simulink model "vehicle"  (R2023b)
settings: Solver=ode3  StartTime=0.0  StopTime=t_end  FixedStep=dt8dof  RelTol=1e-3
PreLoadFcn:
  | define_swarm_buses(3, 1000);
model workspace (MAT data in the model file):
  Af = 1.8
  Cp_tyre = 500
  Cx = 0.28
  G = 15000
  Ha = 0.4
  Hg = 0.4
  Hroll = 0.304
  Hroll_f = 0.08
  Hroll_r = 0.12
  Ir = 0.8
  Ix = 450
  Jz = 1800
  K = 130000
  K_psi = 0.48
  K_y = 0.06
  Karb_F = 26000
  Karb_R = 26000
  KdF = 0
  KdR = 0
  Kd_h = 0
  Kd_v = 0
  Kd_y = 0
  Ki_h = 0
  Ki_v = 0.1
  Ki_y = 0
  Kp_h = 1.5
  Kp_v = 1.5
  Kp_y = 0.1
  Ks_f = 39000
  Ks_r = 39000
  Kv = 290000
  L = 1.5
  Lril_L = 0.055
  Lril_T = 0.5
  MAX_PATH_LEN = 1000
  Pacn = [3000 1 1 1 1 1 1 1 1 0 0 0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]
  R0 = 0.2
  Rfront = 0.2
  Rr_sterzo = 0
  Rrear = 0.2
  Rs = 13
  Tf = 1.5
  Tr = 1.5
  a = 0.6
  a_brake = -3
  b = 0.9
  camb_0F = 0
  camb_0R = -0.00680678408278
  d_max = 0.558505360638
  dt8dof = 0.002
  dtastar = 0.1
  dtcontrol = 0.03
  f0 = 0.0041
  f2 = 2.051e-07
  g = 9.81
  m = 1300
  mot_T_table = [0 0 0 0 0 0 0 0 0 0 0 0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]
  mot_alpha_bp = [0 10 20 30 40 50 60 70 80 90 100]
  mot_n_bp = [0 29.9163426864 59.8326853729 89.7490280593 119.665370746 149.581713432 179.498056119 209.414398805 239.330741492 269.247084178 299.163426864 329.079769551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]
  mpc_speed : object (value not decoded)
  phi_road0 = 0
  psi0 = 0
  r_goal = 5
  r_slow = 30
  replan_steps = 20
  rho = 1.3
  slope_x_body0 = 0
  slope_y_body0 = 0
  t_end = 70
  terrain_truth_mu_table = [-1 -1 -1 -1 -1 -1 -1 -1 -1 -1 -1 -1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]
  terrain_truth_obstacle_table = [1 1 1 1 1 1 1 1 1 1 1 1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]
  terrain_truth_slope_deg_table = [2.67415653197 2.67413215857 2.67406695826 2.6739952249 2.6739164067 2.67382991742 2.67373513563 2.67363140411 2.67351802953 2.67339428225 2.67325939642 2.67311257041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]
  terrain_truth_slope_x_table = [-0.0458815772305 -0.0458808922252 -0.0458794511544 -0.0458778616187 -0.0458761104845 -0.0458741837099 -0.0458720663111 -0.0458697423295 -0.0458671948025 -0.0458644057365 -0.0458613560839 -0.045858025724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]
  terrain_truth_slope_y_table = [0.00874081815183 0.00874213563744 0.00874360556 0.00874524373283 0.00874706738108 0.00874909524079 0.00875134766185 0.00875384671474 0.00875661630067 0.00875968226488 0.00876307251276 0.0087668171283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]
  terrain_truth_traversable_table = [0 0 0 0 0 0 0 0 0 0 0 0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]
  terrain_truth_x_bp = [0 1 2 3 4 5 6 7 8 9 10 11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]
  terrain_truth_y_bp = [0 1 2 3 4 5 6 7 8 9 10 11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]
  teta0 = 0
  tetapunto0 = 0
  theta_road0 = 0
  toe_F = -0.00174532925199
  toe_R = 0.00174532925199
  velstart = 5
  wr0_FL = 3.15
  wr0_FR = 3.15
  wr0_RL = 3.15
  wr0_RR = 3.15
  x0 = 0
  y0 = 0
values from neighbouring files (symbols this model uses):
  gear_ratio = 10    [motor_map.m]
  v_ref_init = scenario.vehicle8.velstart    [make_vref_filter.m]
undefined symbols (not defined in the file or in its folder): A_f, B_f, C_f, D_f, psi0_1
libraries: simulink_extras x15, mpclib x1, slpidlib x1
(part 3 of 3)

== matlab function vehicle/PLANT/VEHICLE 8DOF/Interazione 
Pneumatici-Terreno/Pneumatico FR/Calcolo FORZA LATERALE & LONGITUDINALE
(Pneumatico - Terreno)/Pacejka 96 ==
function [F_pac,C_F] = fcn(Pac,gamma,slip,alfa,Fz,mu,Vcx,R0)
% function x il calcolo delle forze Fx, Fy e Mz

% Pac   -> struttura con coeff. Pacejka 96
% slip     -> scorrimento
% alfa  -> deriva [rad]
% gamma -> camber [rad]
% Vcx,y componenti della velocita' del centro di contatto C della ruota

% Ricostruzione struttura: coefficienti modello 
Pa_FZ0_ = Pac(1);
Pa_LFZ0 = Pac(2);
Pa_LmuV = Pac(3);
Pa_LKXK = Pac(4);
Pa_LKYA = Pac(5);
Pa_LCX_ = Pac(6);
Pa_LCY_ = Pac(7);
Pa_LEX_ = Pac(8);
Pa_LEY_ = Pac(9);
Pa_LHX_ = Pac(10);
Pa_LHY_ = Pac(11);
Pa_LVX_ = Pac(12);
Pa_LVY_ = Pac(13);
Pa_LKYG = Pac(14);
Pa_LKZG = Pac(15);
Pa_LT__ = Pac(16);
Pa_MR__ = Pac(17);
Pa_LXA_ = Pac(18);
Pa_LYK_ = Pac(19);
Pa_LVYK = Pac(20);
Pa_LS__ = Pac(21);
Pa_LCZ_ = Pac(22);
Pa_LMX_ = Pac(23);
Pa_LMY_ = Pac(24);
Pa_PCX1 = Pac(25);
Pa_PDX1 = Pac(26);
Pa_PDX2 = Pac(27);
Pa_PEX1 = Pac(28);
Pa_PEX2 = Pac(29);
Pa_PEX3 = Pac(30);
Pa_PEX4 = Pac(31);
Pa_PKX1 = Pac(32);
Pa_PKX2 = Pac(33);
Pa_PKX3 = Pac(34);
Pa_PHX1 = Pac(35);
Pa_PHX2 = Pac(36);
Pa_PVX1 = Pac(37);
Pa_PVX2 = Pac(38);
Pa_RBX1 = Pac(39);
Pa_RBX2 = Pac(40);
Pa_RCX1 = Pac(41);
Pa_RHX1 = Pac(42);
Pa_RTX1 = Pac(43);
Pa_RTX2 = Pac(44);
Pa_RTX3 = Pac(45);
Pa_QSX1 = Pac(46);
Pa_QSX2 = Pac(47);
Pa_QSX3 = Pac(48);
Pa_PCY1 = Pac(49);
Pa_PDY1 = Pac(50);
Pa_PDY2 = Pac(51);
Pa_PDY3 = Pac(52);
Pa_PEY1 = Pac(53);
Pa_PEY2 = Pac(54);
Pa_PEY3 = Pac(55);
Pa_PEY4 = Pac(56);
Pa_PKY1 = Pac(57);
Pa_PKY2 = Pac(58);
Pa_PKY3 = Pac(59);
Pa_PHY1 = Pac(60);
Pa_PHY2 = Pac(61);
Pa_PHY3 = Pac(62);
Pa_PVY1 = Pac(63);
Pa_PVY2 = Pac(64);
Pa_PVY3 = Pac(65);
Pa_PVY4 = Pac(66);
Pa_RBY1 = Pac(67);
Pa_RBY2 = Pac(68);
Pa_RBY3 = Pac(69);
Pa_RCY1 = Pac(70);
Pa_RHY1 = Pac(71);
Pa_RVY1 = Pac(72);
Pa_RVY2 = Pac(73);
Pa_RVY3 = Pac(74);
Pa_RVY4 = Pac(75);
Pa_RVY5 = Pac(76);
Pa_RVY6 = Pac(77);
Pa_PTY1 = Pac(78);
Pa_PTY2 = Pac(79);
Pa_QSY1 = Pac(80);
Pa_QSY2 = Pac(81);
Pa_QBZ1 = Pac(82);
Pa_QBZ2 = Pac(83);
Pa_QBZ3 = Pac(84);
Pa_QBZ4 = Pac(85);
Pa_QBZ5 = Pac(86);
Pa_QBZ6 = Pac(87);
Pa_QBZ9 = Pac(88);
Pa_QBZZ = Pac(89);
Pa_QCZ1 = Pac(90);
Pa_QDZ1 = Pac(91);
Pa_QDZ2 = Pac(92);
Pa_QDZ3 = Pac(93);
Pa_QDZ4 = Pac(94);
Pa_QDZ6 = Pac(95);
Pa_QDZ7 = Pac(96);
Pa_QDZ8 = Pac(97);
Pa_QDZ9 = Pac(98);
Pa_QEZ1 = Pac(99);
Pa_QEZ2 = Pac(100);
Pa_QEZ3 = Pac(101);
Pa_QEZ4 = Pac(102);
Pa_QEZ5 = Pac(103);
Pa_QHZ1 = Pac(104);
Pa_QHZ2 = Pac(105);
Pa_QHZ3 = Pac(106);
Pa_QHZ4 = Pac(107);
Pa_SSZ1 = Pac(108);
Pa_SSZ2 = Pac(109);
Pa_SSZ3 = Pac(110);
Pa_SSZ4 = Pac(111);
Pa_QTZ1 = Pac(112);

% Costanti
epsi = 0.01;
eps_V = 0.1;
csi_0=1;
csi_4=1;
Amu = 10;
Pa_LmuX = mu;
Pa_LmuY = mu;

%-------------------------------- Fx pure slip ---------------------------
Cx = Pa_PCX1*Pa_LCX_;
dfz = (Fz-Pa_LFZ0*Pa_FZ0_)/(Pa_LFZ0*Pa_FZ0_);
mux = Pa_LmuX * (Pa_PDX1 + Pa_PDX2 * dfz);
Dx = mux*Fz; %*csi_1, con csi_1=1
%Shx = (Pa_PHX1+Pa_PHX2*dfz)*Pa_LHX_;
Shx = 0;
Kx = slip + Shx;
Ex = (Pa_PEX1+Pa_PEX2*dfz+Pa_PEX3*dfz^2)*(1-Pa_PEX4*sign(Kx))*Pa_LEX_;
if Ex>1 Et=1; end
Kxk = Fz*(Pa_PKX1+Pa_PKX2*dfz)*exp(Pa_PKX3*dfz)*Pa_LKXK;
Bx = Kxk/(Cx*Dx+epsi);
lam_mux  = Pa_LmuX*Amu/(1+(Amu-1)*Pa_LmuX);
SVx = Fz*(Pa_PVX1+Pa_PVX2*dfz)*(abs(Vcx)/(abs(Vcx)+eps_V))*Pa_LVX_*lam_mux; %*csi_1, con csi_1=1

% logitudinal slip stiffness (pendenza curva Fx nell'origine)
C_Fk = Bx*Cx*Dx;

% Forza longitudinale
Fx0 = Dx*sin(Cx*atan(Bx*Kx-Ex*(Bx*Kx-atan(Bx*Kx)))) + SVx;

%---------------------------- Fy pure side slip --------------------------
seg=sign(Vcx);
if seg==0 seg=1; end
alfa_star = tan(alfa)*seg;
gam_star = sin(gamma);
Shy = (Pa_PHY1+Pa_PHY2*dfz)*Pa_LHY_+Pa_PHY3*gam_star*Pa_LKYG*csi_0+csi_4-1;
alfa_y = alfa_star + Shy;
Cy = Pa_PCY1*Pa_LCY_;
muy = Pa_LmuY*(Pa_PDY1+Pa_PDY2*dfz)*(1-Pa_PDY3*gam_star^2);
Dy = muy*Fz; %*csi_2, con csi_2=1
Ey = (Pa_PEY1+Pa_PEY2*dfz)*(1-(Pa_PEY3+Pa_PEY4*gam_star)*sign(alfa_y))*Pa_LEY_;
if Ey>1 Ey=1; end
Kya0 = Pa_PKY1*Pa_LFZ0*Pa_FZ0_*sin(2*atan(Fz/(Pa_PKY2*Pa_LFZ0*Pa_FZ0_)))*Pa_LKYA;
Kya = Kya0*(1-Pa_PKY3*gam_star^2); %*csi_3, con csi_3=1
By = Kya/(Cy*Dy+epsi);
lam_muy = Pa_LmuY*Amu/(1+(Amu-1)*Pa_LmuY);
SVy = Fz*((Pa_PVY1+Pa_PVY2*dfz)*Pa_LVY_+(Pa_PVY3+Pa_PVY4*dfz)*gam_star*Pa_LKYG )*lam_muy; %*csi_2, con csi_2=1
Kyg0 = (Pa_PHY3*Kya0+Fz*(Pa_PVY3+Pa_PVY4*dfz))*Pa_LKYG;

% cornering stiffness (pendenza curva Fy nell'origine)
C_Fa = By*Cy*Dy;

% Forza laterale
Fy0 = Dy*sin(Cy*atan(By*alfa_y-Ey*(By*alfa_y-atan(By*alfa_y)))) + SVy;

% --------------------- Fx combined slip ------------------------------
Shxa = Pa_RHX1;
%Exa = Pa_REX1+Pa_REX2*dfz; NON esiste Pa.REX1 ne' Pa.REX2
Exa = 0;
Cxa = Pa_RCX1;
Bxa = Pa_RBX1*cos(atan(Pa_RBX2*slip))*Pa_LXA_;
alfaS = alfa_star+Shxa;
Gxa0 = cos(Cxa*atan(Bxa*Shxa-Exa*(Bxa*Shxa-atan(Bxa*Shxa))));
Gxa = cos(Cxa*atan(Bxa*alfaS-Exa*(Bxa*alfaS-atan(Bxa*alfaS))))/Gxa0;
Fx = Fx0*Gxa;

% ---------------------- Fy combined slip ------------------------------
Dvyk = muy*Fz*(Pa_RVY1+Pa_RVY2*dfz+Pa_RVY3*gam_star)*cos(atan(Pa_RVY4*alfa_star));%*csi_2, con csi_2=1
Svyk = Dvyk*sin(Pa_RVY5*atan(Pa_RVY6*slip));
Shyk = Pa_RHY1; %+Pa.RHY2*dfz; NON esiste Pa.RHY2
Cyk = Pa_RCY1;
Byk = Pa_RBY1*cos(atan(Pa_RBY2*(alfa_star-Pa_RBY3)))*Pa_LYK_;
%Eyk = Pa_REY1+Pa_REY2*dfz; NON esiste Pa.REY1 ne' Pa.REY2
Eyk = 0;
ks = slip+Shyk;
Gyk0 = cos(Cyk*atan(Byk*Shyk-Eyk*(Byk*Shyk-atan(Byk*Shyk))));
Gyk = cos(Cyk*atan(Byk*ks-Eyk*(Byk*ks-atan(Byk*ks))))/Gyk0;
Fy = Fy0*Gyk+Svyk;

% --------------------- Mz pure side slip  ---------------------------
Shf = Shy+SVy/Kya;
alfa_r = alfa_star+Shf;
Br = (Pa_QBZ9/Pa_LmuY+Pa_QBZZ*By*Cy); %*csi_6, con csi_6=1
%%% Pa_QBZZ e' in realta' QBZ10 scritto cosi' x ragioni di spazio
Cr = 1; %*csi_7, con csi_7=1
Dr = Fz*R0*((Pa_QDZ6+Pa_QDZ7*dfz)+(Pa_QDZ8+Pa_QDZ9*dfz)*gam_star)*cos(alfa)*Pa_LmuY*seg; %+csi_8-1, con csi_8=1
Mzr0 = Dr*cos(Cr*atan(Br*alfa_r));
Sht = Pa_QHZ1+Pa_QHZ2*dfz+(Pa_QHZ3+Pa_QHZ4*dfz)*gam_star;
alfa_t = alfa_star+Sht;
Bt = (Pa_QBZ1+Pa_QBZ2*dfz+Pa_QBZ3*dfz^2)*(1+Pa_QBZ5*abs(gam_star)+Pa_QBZ6*gam_star^2)*Pa_LKYA/Pa_LmuY;
if Bt<0 Bt=0; end
Ct = Pa_QCZ1;
Dt0 = Fz*R0/(Pa_LFZ0*Pa_FZ0_)*(Pa_QDZ1+Pa_QDZ2*dfz)*seg;
Dt = Dt0*(1+Pa_QDZ3*abs(gam_star)+Pa_QDZ4*gam_star^2); %*csi_5, con csi_5=1
Et = (Pa_QEZ1+Pa_QEZ2*dfz+Pa_QEZ3*dfz^2)*(1+(Pa_QEZ4+Pa_QEZ5*gam_star)*2/pi*atan(Bt*Ct*alfa_t));
if Et>1 Et=1; end
t0 = Dt*cos(Ct*atan(Bt*alfa_t - Et*(Bt*alfa_t-atan(Bt*alfa_t))))*cos(alfa);
Mz0 = -t0*Fy;
Kza0 = Dt0*Kya0;
%Kzg0 = Fz*R0*(Pa_QDZ8+Pa_QDZ9*dfz)-Dt0*Kyg0;

% momento autoallineamento (aligning torque)
Mz = Mz0 + Mzr0;

% ------------------------ Mz Combined -----------------------------
eps_k = 0; % ???????
lambda_s = Pa_LS__ ;
Fz0p = Pa_LFZ0*Pa_FZ0_;
K_yap = Kya + eps_k;
alfa_req = sqrt(alfa_r^2+(Kxk/K_yap)^2*slip^2)*sign(alfa_r);
alfa_teq = sqrt(alfa_t^2+(Kxk/K_yap)^2*slip^2)*sign(alfa_t);
s = R0*(Pa_SSZ1 + Pa_SSZ2*(Fy/Fz0p) + (Pa_SSZ3+Pa_SSZ4*dfz)*gam_star)*lambda_s;
Mzr = Dr*cos(Cr*atan(Br*alfa_req));
Fyp = Fy-Svyk; 
t = Dt*cos(Ct*atan(Bt*alfa_teq - Et*(Bt*alfa_teq-atan(Bt*alfa_teq))))*cos(alfa);
Mzp = -t*Fyp;
% momento autoallineamento (aligning torque)
Mz = Mzp + Mzr + s*Fx;
%%%%%%%%%%%%%%%%%%%%%%%

% Controllo che forza verticale Fz sia positiva
if Fz <= 0
    Fx = 0;
    Fy = 0;
    Mz = 0;
end

% Output
F_pac = [Fx; Fy; Mz];
C_F = [C_Fk; C_Fa];

== matlab function vehicle/PLANT/VEHICLE 8DOF/Interazione 
Pneumatici-Terreno/Pneumatico RL/Calcolo FORZA LATERALE & LONGITUDINALE
(Pneumatico - Terreno)/Pacejka 96 ==
function [F_pac,C_F] = fcn(Pac,gamma,slip,alfa,Fz,mu,Vcx,R0)
% function x il calcolo delle forze Fx, Fy e Mz

% Pac   -> struttura con coeff. Pacejka 96
% slip     -> scorrimento
% alfa  -> deriva [rad]
% gamma -> camber [rad]
% Vcx,y componenti della velocita' del centro di contatto C della ruota

% Ricostruzione struttura: coefficienti modello 
Pa_FZ0_ = Pac(1);
Pa_LFZ0 = Pac(2);
Pa_LmuV = Pac(3);
Pa_LKXK = Pac(4);
Pa_LKYA = Pac(5);
Pa_LCX_ = Pac(6);
Pa_LCY_ = Pac(7);
Pa_LEX_ = Pac(8);
Pa_LEY_ = Pac(9);
Pa_LHX_ = Pac(10);
Pa_LHY_ = Pac(11);
Pa_LVX_ = Pac(12);
Pa_LVY_ = Pac(13);
Pa_LKYG = Pac(14);
Pa_LKZG = Pac(15);
Pa_LT__ = Pac(16);
Pa_MR__ = Pac(17);
Pa_LXA_ = Pac(18);
Pa_LYK_ = Pac(19);
Pa_LVYK = Pac(20);
Pa_LS__ = Pac(21);
Pa_LCZ_ = Pac(22);
Pa_LMX_ = Pac(23);
Pa_LMY_ = Pac(24);
Pa_PCX1 = Pac(25);
Pa_PDX1 = Pac(26);
Pa_PDX2 = Pac(27);
Pa_PEX1 = Pac(28);
Pa_PEX2 = Pac(29);
Pa_PEX3 = Pac(30);
Pa_PEX4 = Pac(31);
Pa_PKX1 = Pac(32);
Pa_PKX2 = Pac(33);
Pa_PKX3 = Pac(34);
Pa_PHX1 = Pac(35);
Pa_PHX2 = Pac(36);
Pa_PVX1 = Pac(37);
Pa_PVX2 = Pac(38);
Pa_RBX1 = Pac(39);
Pa_RBX2 = Pac(40);
Pa_RCX1 = Pac(41);
Pa_RHX1 = Pac(42);
Pa_RTX1 = Pac(43);
Pa_RTX2 = Pac(44);
Pa_RTX3 = Pac(45);
Pa_QSX1 = Pac(46);
Pa_QSX2 = Pac(47);
Pa_QSX3 = Pac(48);
Pa_PCY1 = Pac(49);
Pa_PDY1 = Pac(50);
Pa_PDY2 = Pac(51);
Pa_PDY3 = Pac(52);
Pa_PEY1 = Pac(53);
Pa_PEY2 = Pac(54);
Pa_PEY3 = Pac(55);
Pa_PEY4 = Pac(56);
Pa_PKY1 = Pac(57);
Pa_PKY2 = Pac(58);
Pa_PKY3 = Pac(59);
Pa_PHY1 = Pac(60);
Pa_PHY2 = Pac(61);
Pa_PHY3 = Pac(62);
Pa_PVY1 = Pac(63);
Pa_PVY2 = Pac(64);
Pa_PVY3 = Pac(65);
Pa_PVY4 = Pac(66);
Pa_RBY1 = Pac(67);
Pa_RBY2 = Pac(68);
Pa_RBY3 = Pac(69);
Pa_RCY1 = Pac(70);
Pa_RHY1 = Pac(71);
Pa_RVY1 = Pac(72);
Pa_RVY2 = Pac(73);
Pa_RVY3 = Pac(74);
Pa_RVY4 = Pac(75);
Pa_RVY5 = Pac(76);
Pa_RVY6 = Pac(77);
Pa_PTY1 = Pac(78);
Pa_PTY2 = Pac(79);
Pa_QSY1 = Pac(80);
Pa_QSY2 = Pac(81);
Pa_QBZ1 = Pac(82);
Pa_QBZ2 = Pac(83);
Pa_QBZ3 = Pac(84);
Pa_QBZ4 = Pac(85);
Pa_QBZ5 = Pac(86);
Pa_QBZ6 = Pac(87);
Pa_QBZ9 = Pac(88);
Pa_QBZZ = Pac(89);
Pa_QCZ1 = Pac(90);
Pa_QDZ1 = Pac(91);
Pa_QDZ2 = Pac(92);
Pa_QDZ3 = Pac(93);
Pa_QDZ4 = Pac(94);
Pa_QDZ6 = Pac(95);
Pa_QDZ7 = Pac(96);
Pa_QDZ8 = Pac(97);
Pa_QDZ9 = Pac(98);
Pa_QEZ1 = Pac(99);
Pa_QEZ2 = Pac(100);
Pa_QEZ3 = Pac(101);
Pa_QEZ4 = Pac(102);
Pa_QEZ5 = Pac(103);
Pa_QHZ1 = Pac(104);
Pa_QHZ2 = Pac(105);
Pa_QHZ3 = Pac(106);
Pa_QHZ4 = Pac(107);
Pa_SSZ1 = Pac(108);
Pa_SSZ2 = Pac(109);
Pa_SSZ3 = Pac(110);
Pa_SSZ4 = Pac(111);
Pa_QTZ1 = Pac(112);

% Costanti
epsi = 0.01;
eps_V = 0.1;
csi_0=1;
csi_4=1;
Amu = 10;
Pa_LmuX = mu;
Pa_LmuY = mu;

%-------------------------------- Fx pure slip ---------------------------
Cx = Pa_PCX1*Pa_LCX_;
dfz = (Fz-Pa_LFZ0*Pa_FZ0_)/(Pa_LFZ0*Pa_FZ0_);
mux = Pa_LmuX * (Pa_PDX1 + Pa_PDX2 * dfz);
Dx = mux*Fz; %*csi_1, con csi_1=1
%Shx = (Pa_PHX1+Pa_PHX2*dfz)*Pa_LHX_;
Shx = 0;
Kx = slip + Shx;
Ex = (Pa_PEX1+Pa_PEX2*dfz+Pa_PEX3*dfz^2)*(1-Pa_PEX4*sign(Kx))*Pa_LEX_;
if Ex>1 Et=1; end
Kxk = Fz*(Pa_PKX1+Pa_PKX2*dfz)*exp(Pa_PKX3*dfz)*Pa_LKXK;
Bx = Kxk/(Cx*Dx+epsi);
lam_mux  = Pa_LmuX*Amu/(1+(Amu-1)*Pa_LmuX);
SVx = Fz*(Pa_PVX1+Pa_PVX2*dfz)*(abs(Vcx)/(abs(Vcx)+eps_V))*Pa_LVX_*lam_mux; %*csi_1, con csi_1=1

% logitudinal slip stiffness (pendenza curva Fx nell'origine)
C_Fk = Bx*Cx*Dx;

% Forza longitudinale
Fx0 = Dx*sin(Cx*atan(Bx*Kx-Ex*(Bx*Kx-atan(Bx*Kx)))) + SVx;

%---------------------------- Fy pure side slip --------------------------
seg=sign(Vcx);
if seg==0 seg=1; end
alfa_star = tan(alfa)*seg;
gam_star = sin(gamma);
Shy = (Pa_PHY1+Pa_PHY2*dfz)*Pa_LHY_+Pa_PHY3*gam_star*Pa_LKYG*csi_0+csi_4-1;
alfa_y = alfa_star + Shy;
Cy = Pa_PCY1*Pa_LCY_;
muy = Pa_LmuY*(Pa_PDY1+Pa_PDY2*dfz)*(1-Pa_PDY3*gam_star^2);
Dy = muy*Fz; %*csi_2, con csi_2=1
Ey = (Pa_PEY1+Pa_PEY2*dfz)*(1-(Pa_PEY3+Pa_PEY4*gam_star)*sign(alfa_y))*Pa_LEY_;
if Ey>1 Ey=1; end
Kya0 = Pa_PKY1*Pa_LFZ0*Pa_FZ0_*sin(2*atan(Fz/(Pa_PKY2*Pa_LFZ0*Pa_FZ0_)))*Pa_LKYA;
Kya = Kya0*(1-Pa_PKY3*gam_star^2); %*csi_3, con csi_3=1
By = Kya/(Cy*Dy+epsi);
lam_muy = Pa_LmuY*Amu/(1+(Amu-1)*Pa_LmuY);
SVy = Fz*((Pa_PVY1+Pa_PVY2*dfz)*Pa_LVY_+(Pa_PVY3+Pa_PVY4*dfz)*gam_star*Pa_LKYG )*lam_muy; %*csi_2, con csi_2=1
Kyg0 = (Pa_PHY3*Kya0+Fz*(Pa_PVY3+Pa_PVY4*dfz))*Pa_LKYG;

% cornering stiffness (pendenza curva Fy nell'origine)
C_Fa = By*Cy*Dy;

% Forza laterale
Fy0 = Dy*sin(Cy*atan(By*alfa_y-Ey*(By*alfa_y-atan(By*alfa_y)))) + SVy;

% --------------------- Fx combined slip ------------------------------
Shxa = Pa_RHX1;
%Exa = Pa_REX1+Pa_REX2*dfz; NON esiste Pa.REX1 ne' Pa.REX2
Exa = 0;
Cxa = Pa_RCX1;
Bxa = Pa_RBX1*cos(atan(Pa_RBX2*slip))*Pa_LXA_;
alfaS = alfa_star+Shxa;
Gxa0 = cos(Cxa*atan(Bxa*Shxa-Exa*(Bxa*Shxa-atan(Bxa*Shxa))));
Gxa = cos(Cxa*atan(Bxa*alfaS-Exa*(Bxa*alfaS-atan(Bxa*alfaS))))/Gxa0;
Fx = Fx0*Gxa;

% ---------------------- Fy combined slip ------------------------------
Dvyk = muy*Fz*(Pa_RVY1+Pa_RVY2*dfz+Pa_RVY3*gam_star)*cos(atan(Pa_RVY4*alfa_star));%*csi_2, con csi_2=1
Svyk = Dvyk*sin(Pa_RVY5*atan(Pa_RVY6*slip));
Shyk = Pa_RHY1; %+Pa.RHY2*dfz; NON esiste Pa.RHY2
Cyk = Pa_RCY1;
Byk = Pa_RBY1*cos(atan(Pa_RBY2*(alfa_star-Pa_RBY3)))*Pa_LYK_;
%Eyk = Pa_REY1+Pa_REY2*dfz; NON esiste Pa.REY1 ne' Pa.REY2
Eyk = 0;
ks = slip+Shyk;
Gyk0 = cos(Cyk*atan(Byk*Shyk-Eyk*(Byk*Shyk-atan(Byk*Shyk))));
Gyk = cos(Cyk*atan(Byk*ks-Eyk*(Byk*ks-atan(Byk*ks))))/Gyk0;
Fy = Fy0*Gyk+Svyk;

% --------------------- Mz pure side slip  ---------------------------
Shf = Shy+SVy/Kya;
alfa_r = alfa_star+Shf;
Br = (Pa_QBZ9/Pa_LmuY+Pa_QBZZ*By*Cy); %*csi_6, con csi_6=1
%%% Pa_QBZZ e' in realta' QBZ10 scritto cosi' x ragioni di spazio
Cr = 1; %*csi_7, con csi_7=1
Dr = Fz*R0*((Pa_QDZ6+Pa_QDZ7*dfz)+(Pa_QDZ8+Pa_QDZ9*dfz)*gam_star)*cos(alfa)*Pa_LmuY*seg; %+csi_8-1, con csi_8=1
Mzr0 = Dr*cos(Cr*atan(Br*alfa_r));
Sht = Pa_QHZ1+Pa_QHZ2*dfz+(Pa_QHZ3+Pa_QHZ4*dfz)*gam_star;
alfa_t = alfa_star+Sht;
Bt = (Pa_QBZ1+Pa_QBZ2*dfz+Pa_QBZ3*dfz^2)*(1+Pa_QBZ5*abs(gam_star)+Pa_QBZ6*gam_star^2)*Pa_LKYA/Pa_LmuY;
if Bt<0 Bt=0; end
Ct = Pa_QCZ1;
Dt0 = Fz*R0/(Pa_LFZ0*Pa_FZ0_)*(Pa_QDZ1+Pa_QDZ2*dfz)*seg;
Dt = Dt0*(1+Pa_QDZ3*abs(gam_star)+Pa_QDZ4*gam_star^2); %*csi_5, con csi_5=1
Et = (Pa_QEZ1+Pa_QEZ2*dfz+Pa_QEZ3*dfz^2)*(1+(Pa_QEZ4+Pa_QEZ5*gam_star)*2/pi*atan(Bt*Ct*alfa_t));
if Et>1 Et=1; end
t0 = Dt*cos(Ct*atan(Bt*alfa_t - Et*(Bt*alfa_t-atan(Bt*alfa_t))))*cos(alfa);
Mz0 = -t0*Fy;
Kza0 = Dt0*Kya0;
%Kzg0 = Fz*R0*(Pa_QDZ8+Pa_QDZ9*dfz)-Dt0*Kyg0;

% momento autoallineamento (aligning torque)
Mz = Mz0 + Mzr0;

% ------------------------ Mz Combined -----------------------------
eps_k = 0; % ???????
lambda_s = Pa_LS__ ;
Fz0p = Pa_LFZ0*Pa_FZ0_;
K_yap = Kya + eps_k;
alfa_req = sqrt(alfa_r^2+(Kxk/K_yap)^2*slip^2)*sign(alfa_r);
alfa_teq = sqrt(alfa_t^2+(Kxk/K_yap)^2*slip^2)*sign(alfa_t);
s = R0*(Pa_SSZ1 + Pa_SSZ2*(Fy/Fz0p) + (Pa_SSZ3+Pa_SSZ4*dfz)*gam_star)*lambda_s;
Mzr = Dr*cos(Cr*atan(Br*alfa_req));
Fyp = Fy-Svyk; 
t = Dt*cos(Ct*atan(Bt*alfa_teq - Et*(Bt*alfa_teq-atan(Bt*alfa_teq))))*cos(alfa);
Mzp = -t*Fyp;
% momento autoallineamento (aligning torque)
Mz = Mzp + Mzr + s*Fx;
%%%%%%%%%%%%%%%%%%%%%%%

% Controllo che forza verticale Fz sia positiva
if Fz <= 0
    Fx = 0;
    Fy = 0;
    Mz = 0;
end

% Output
F_pac = [Fx; Fy; Mz];
C_F = [C_Fk; C_Fa];

== matlab function vehicle/PLANT/VEHICLE 8DOF/Interazione 
Pneumatici-Terreno/Pneumatico RR/Calcolo FORZA LATERALE & LONGITUDINALE
(Pneumatico - Terreno)/Pacejka 96 ==
function [F_pac,C_F] = fcn(Pac,gamma,slip,alfa,Fz,mu,Vcx,R0)
% function x il calcolo delle forze Fx, Fy e Mz

% Pac   -> struttura con coeff. Pacejka 96
% slip     -> scorrimento
% alfa  -> deriva [rad]
% gamma -> camber [rad]
% Vcx,y componenti della velocita' del centro di contatto C della ruota

% Ricostruzione struttura: coefficienti modello 
Pa_FZ0_ = Pac(1);
Pa_LFZ0 = Pac(2);
Pa_LmuV = Pac(3);
Pa_LKXK = Pac(4);
Pa_LKYA = Pac(5);
Pa_LCX_ = Pac(6);
Pa_LCY_ = Pac(7);
Pa_LEX_ = Pac(8);
Pa_LEY_ = Pac(9);
Pa_LHX_ = Pac(10);
Pa_LHY_ = Pac(11);
Pa_LVX_ = Pac(12);
Pa_LVY_ = Pac(13);
Pa_LKYG = Pac(14);
Pa_LKZG = Pac(15);
Pa_LT__ = Pac(16);
Pa_MR__ = Pac(17);
Pa_LXA_ = Pac(18);
Pa_LYK_ = Pac(19);
Pa_LVYK = Pac(20);
Pa_LS__ = Pac(21);
Pa_LCZ_ = Pac(22);
Pa_LMX_ = Pac(23);
Pa_LMY_ = Pac(24);
Pa_PCX1 = Pac(25);
Pa_PDX1 = Pac(26);
Pa_PDX2 = Pac(27);
Pa_PEX1 = Pac(28);
Pa_PEX2 = Pac(29);
Pa_PEX3 = Pac(30);
Pa_PEX4 = Pac(31);
Pa_PKX1 = Pac(32);
Pa_PKX2 = Pac(33);
Pa_PKX3 = Pac(34);
Pa_PHX1 = Pac(35);
Pa_PHX2 = Pac(36);
Pa_PVX1 = Pac(37);
Pa_PVX2 = Pac(38);
Pa_RBX1 = Pac(39);
Pa_RBX2 = Pac(40);
Pa_RCX1 = Pac(41);
Pa_RHX1 = Pac(42);
Pa_RTX1 = Pac(43);
Pa_RTX2 = Pac(44);
Pa_RTX3 = Pac(45);
Pa_QSX1 = Pac(46);
Pa_QSX2 = Pac(47);
Pa_QSX3 = Pac(48);
Pa_PCY1 = Pac(49);
Pa_PDY1 = Pac(50);
Pa_PDY2 = Pac(51);
Pa_PDY3 = Pac(52);
Pa_PEY1 = Pac(53);
Pa_PEY2 = Pac(54);
Pa_PEY3 = Pac(55);
Pa_PEY4 = Pac(56);
Pa_PKY1 = Pac(57);
Pa_PKY2 = Pac(58);
Pa_PKY3 = Pac(59);
Pa_PHY1 = Pac(60);
Pa_PHY2 = Pac(61);
Pa_PHY3 = Pac(62);
Pa_PVY1 = Pac(63);
Pa_PVY2 = Pac(64);
Pa_PVY3 = Pac(65);
Pa_PVY4 = Pac(66);
Pa_RBY1 = Pac(67);
Pa_RBY2 = Pac(68);
Pa_RBY3 = Pac(69);
Pa_RCY1 = Pac(70);
Pa_RHY1 = Pac(71);
Pa_RVY1 = Pac(72);
Pa_RVY2 = Pac(73);
Pa_RVY3 = Pac(74);
Pa_RVY4 = Pac(75);
Pa_RVY5 = Pac(76);
Pa_RVY6 = Pac(77);
Pa_PTY1 = Pac(78);
Pa_PTY2 = Pac(79);
Pa_QSY1 = Pac(80);
Pa_QSY2 = Pac(81);
Pa_QBZ1 = Pac(82);
Pa_QBZ2 = Pac(83);
Pa_QBZ3 = Pac(84);
Pa_QBZ4 = Pac(85);
Pa_QBZ5 = Pac(86);
Pa_QBZ6 = Pac(87);
Pa_QBZ9 = Pac(88);
Pa_QBZZ = Pac(89);
Pa_QCZ1 = Pac(90);
Pa_QDZ1 = Pac(91);
Pa_QDZ2 = Pac(92);
Pa_QDZ3 = Pac(93);
Pa_QDZ4 = Pac(94);
Pa_QDZ6 = Pac(95);
Pa_QDZ7 = Pac(96);
Pa_QDZ8 = Pac(97);
Pa_QDZ9 = Pac(98);
Pa_QEZ1 = Pac(99);
Pa_QEZ2 = Pac(100);
Pa_QEZ3 = Pac(101);
Pa_QEZ4 = Pac(102);
Pa_QEZ5 = Pac(103);
Pa_QHZ1 = Pac(104);
Pa_QHZ2 = Pac(105);
Pa_QHZ3 = Pac(106);
Pa_QHZ4 = Pac(107);
Pa_SSZ1 = Pac(108);
Pa_SSZ2 = Pac(109);
Pa_SSZ3 = Pac(110);
Pa_SSZ4 = Pac(111);
Pa_QTZ1 = Pac(112);

% Costanti
epsi = 0.01;
eps_V = 0.1;
csi_0=1;
csi_4=1;
Amu = 10;
Pa_LmuX = mu;
Pa_LmuY = mu;

%-------------------------------- Fx pure slip ---------------------------
Cx = Pa_PCX1*Pa_LCX_;
dfz = (Fz-Pa_LFZ0*Pa_FZ0_)/(Pa_LFZ0*Pa_FZ0_);
mux = Pa_LmuX * (Pa_PDX1 + Pa_PDX2 * dfz);
Dx = mux*Fz; %*csi_1, con csi_1=1
%Shx = (Pa_PHX1+Pa_PHX2*dfz)*Pa_LHX_;
Shx = 0;
Kx = slip + Shx;
Ex = (Pa_PEX1+Pa_PEX2*dfz+Pa_PEX3*dfz^2)*(1-Pa_PEX4*sign(Kx))*Pa_LEX_;
if Ex>1 Et=1; end
Kxk = Fz*(Pa_PKX1+Pa_PKX2*dfz)*exp(Pa_PKX3*dfz)*Pa_LKXK;
Bx = Kxk/(Cx*Dx+epsi);
lam_mux  = Pa_LmuX*Amu/(1+(Amu-1)*Pa_LmuX);
SVx = Fz*(Pa_PVX1+Pa_PVX2*dfz)*(abs(Vcx)/(abs(Vcx)+eps_V))*Pa_LVX_*lam_mux; %*csi_1, con csi_1=1

% logitudinal slip stiffness (pendenza curva Fx nell'origine)
C_Fk = Bx*Cx*Dx;

% Forza longitudinale
Fx0 = Dx*sin(Cx*atan(Bx*Kx-Ex*(Bx*Kx-atan(Bx*Kx)))) + SVx;

%---------------------------- Fy pure side slip --------------------------
seg=sign(Vcx);
if seg==0 seg=1; end
alfa_star = tan(alfa)*seg;
gam_star = sin(gamma);
Shy = (Pa_PHY1+Pa_PHY2*dfz)*Pa_LHY_+Pa_PHY3*gam_star*Pa_LKYG*csi_0+csi_4-1;
alfa_y = alfa_star + Shy;
Cy = Pa_PCY1*Pa_LCY_;
muy = Pa_LmuY*(Pa_PDY1+Pa_PDY2*dfz)*(1-Pa_PDY3*gam_star^2);
Dy = muy*Fz; %*csi_2, con csi_2=1
Ey = (Pa_PEY1+Pa_PEY2*dfz)*(1-(Pa_PEY3+Pa_PEY4*gam_star)*sign(alfa_y))*Pa_LEY_;
if Ey>1 Ey=1; end
Kya0 = Pa_PKY1*Pa_LFZ0*Pa_FZ0_*sin(2*atan(Fz/(Pa_PKY2*Pa_LFZ0*Pa_FZ0_)))*Pa_LKYA;
Kya = Kya0*(1-Pa_PKY3*gam_star^2); %*csi_3, con csi_3=1
By = Kya/(Cy*Dy+epsi);
lam_muy = Pa_LmuY*Amu/(1+(Amu-1)*Pa_LmuY);
SVy = Fz*((Pa_PVY1+Pa_PVY2*dfz)*Pa_LVY_+(Pa_PVY3+Pa_PVY4*dfz)*gam_star*Pa_LKYG )*lam_muy; %*csi_2, con csi_2=1
Kyg0 = (Pa_PHY3*Kya0+Fz*(Pa_PVY3+Pa_PVY4*dfz))*Pa_LKYG;

% cornering stiffness (pendenza curva Fy nell'origine)
C_Fa = By*Cy*Dy;

% Forza laterale
Fy0 = Dy*sin(Cy*atan(By*alfa_y-Ey*(By*alfa_y-atan(By*alfa_y)))) + SVy;

% --------------------- Fx combined slip ------------------------------
Shxa = Pa_RHX1;
%Exa = Pa_REX1+Pa_REX2*dfz; NON esiste Pa.REX1 ne' Pa.REX2
Exa = 0;
Cxa = Pa_RCX1;
Bxa = Pa_RBX1*cos(atan(Pa_RBX2*slip))*Pa_LXA_;
alfaS = alfa_star+Shxa;
Gxa0 = cos(Cxa*atan(Bxa*Shxa-Exa*(Bxa*Shxa-atan(Bxa*Shxa))));
Gxa = cos(Cxa*atan(Bxa*alfaS-Exa*(Bxa*alfaS-atan(Bxa*alfaS))))/Gxa0;
Fx = Fx0*Gxa;

% ---------------------- Fy combined slip ------------------------------
Dvyk = muy*Fz*(Pa_RVY1+Pa_RVY2*dfz+Pa_RVY3*gam_star)*cos(atan(Pa_RVY4*alfa_star));%*csi_2, con csi_2=1
Svyk = Dvyk*sin(Pa_RVY5*atan(Pa_RVY6*slip));
Shyk = Pa_RHY1; %+Pa.RHY2*dfz; NON esiste Pa.RHY2
Cyk = Pa_RCY1;
Byk = Pa_RBY1*cos(atan(Pa_RBY2*(alfa_star-Pa_RBY3)))*Pa_LYK_;
%Eyk = Pa_REY1+Pa_REY2*dfz; NON esiste Pa.REY1 ne' Pa.REY2
Eyk = 0;
ks = slip+Shyk;
Gyk0 = cos(Cyk*atan(Byk*Shyk-Eyk*(Byk*Shyk-atan(Byk*Shyk))));
Gyk = cos(Cyk*atan(Byk*ks-Eyk*(Byk*ks-atan(Byk*ks))))/Gyk0;
Fy = Fy0*Gyk+Svyk;

% --------------------- Mz pure side slip  ---------------------------
Shf = Shy+SVy/Kya;
alfa_r = alfa_star+Shf;
Br = (Pa_QBZ9/Pa_LmuY+Pa_QBZZ*By*Cy); %*csi_6, con csi_6=1
%%% Pa_QBZZ e' in realta' QBZ10 scritto cosi' x ragioni di spazio
Cr = 1; %*csi_7, con csi_7=1
Dr = Fz*R0*((Pa_QDZ6+Pa_QDZ7*dfz)+(Pa_QDZ8+Pa_QDZ9*dfz)*gam_star)*cos(alfa)*Pa_LmuY*seg; %+csi_8-1, con csi_8=1
Mzr0 = Dr*cos(Cr*atan(Br*alfa_r));
Sht = Pa_QHZ1+Pa_QHZ2*dfz+(Pa_QHZ3+Pa_QHZ4*dfz)*gam_star;
alfa_t = alfa_star+Sht;
Bt = (Pa_QBZ1+Pa_QBZ2*dfz+Pa_QBZ3*dfz^2)*(1+Pa_QBZ5*abs(gam_star)+Pa_QBZ6*gam_star^2)*Pa_LKYA/Pa_LmuY;
if Bt<0 Bt=0; end
Ct = Pa_QCZ1;
Dt0 = Fz*R0/(Pa_LFZ0*Pa_FZ0_)*(Pa_QDZ1+Pa_QDZ2*dfz)*seg;
Dt = Dt0*(1+Pa_QDZ3*abs(gam_star)+Pa_QDZ4*gam_star^2); %*csi_5, con csi_5=1
Et = (Pa_QEZ1+Pa_QEZ2*dfz+Pa_QEZ3*dfz^2)*(1+(Pa_QEZ4+Pa_QEZ5*gam_star)*2/pi*atan(Bt*Ct*alfa_t));
if Et>1 Et=1; end
t0 = Dt*cos(Ct*atan(Bt*alfa_t - Et*(Bt*alfa_t-atan(Bt*alfa_t))))*cos(alfa);
Mz0 = -t0*Fy;
Kza0 = Dt0*Kya0;
%Kzg0 = Fz*R0*(Pa_QDZ8+Pa_QDZ9*dfz)-Dt0*Kyg0;

% momento autoallineamento (aligning torque)
Mz = Mz0 + Mzr0;

% ------------------------ Mz Combined -----------------------------
eps_k = 0; % ???????
lambda_s = Pa_LS__ ;
Fz0p = Pa_LFZ0*Pa_FZ0_;
K_yap = Kya + eps_k;
alfa_req = sqrt(alfa_r^2+(Kxk/K_yap)^2*slip^2)*sign(alfa_r);
alfa_teq = sqrt(alfa_t^2+(Kxk/K_yap)^2*slip^2)*sign(alfa_t);
s = R0*(Pa_SSZ1 + Pa_SSZ2*(Fy/Fz0p) + (Pa_SSZ3+Pa_SSZ4*dfz)*gam_star)*lambda_s;
Mzr = Dr*cos(Cr*atan(Br*alfa_req));
Fyp = Fy-Svyk; 
t = Dt*cos(Ct*atan(Bt*alfa_teq - Et*(Bt*alfa_teq-atan(Bt*alfa_teq))))*cos(alfa);
Mzp = -t*Fyp;
% momento autoallineamento (aligning torque)
Mz = Mzp + Mzr + s*Fx;
%%%%%%%%%%%%%%%%%%%%%%%

% Controllo che forza verticale Fz sia positiva
if Fz <= 0
    Fx = 0;
    Fy = 0;
    Mz = 0;
end

% Output
F_pac = [Fx; Fy; Mz];
C_F = [C_Fk; C_Fa];

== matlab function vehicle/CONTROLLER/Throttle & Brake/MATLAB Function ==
function F_md = md_fluxweak(v_actual, accel_prev, F_res)
%#codegen
% MD aumentata: F_res + "buco" di trazione da flux weakening.
    T_peak_mot = 15; n_mot = 4;            % per motore, n. motori (da motor_map.m)
    P_peak = 7.5e3; gear = 10; R0 = 0.2;
    k_v      = (gear*(n_mot*T_peak_mot)/100)/R0;   % 30 N/%
    v_corner = (P_peak/T_peak_mot)*R0/gear;        % 10 m/s
    phi   = min(1, v_corner/max(v_actual,0.1));
    F_def = k_v*(1-phi)*max(accel_prev,0);         % forza mancante [N]
    F_md  = F_res + F_def;
end
%al posto di questa funzione si può anche usare una lookup table, se un
%giorno si dovesse usare una mappa motore dove P_peak non è costante e il
%flux weakening non è semplicemente un iperbole

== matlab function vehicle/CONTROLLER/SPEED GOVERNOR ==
function [v_ref, v_ref_raw, v_max_global, ...
    v_curve_mu, ...
    v_rollover, ...
    v_goal, ...
    v_unknown, ...
    v_ltr] = SpeedReferenceGovernor( ...
    v_max_global, ...
    V, kappa_next, d_goal, mu_next, angle_long, angle_lat, ...
    Fz_FL, Fz_FR, Fz_RL, Fz_RR, ...
    unknown_ratio_ahead, v_ref_prev, Ts, r_goal)

%#codegen

%% Parametri veicolo
g = 9.81;
T_track = 1.0;      % carreggiata [m] - metti il tuo valore
h_CG = 0.45;        % altezza baricentro [m] - metti il tuo valore

%% Parametri sicurezza
eta_mu = 0.85;
eta_brake = 0.4;
eta_roll = 0.80; %0.8 roll è circa 0.85 mu, il tutto è sovrapposto, cancellare mu e tenere roll, dire che sono equivalenti

kappa_eps = 1e-4;

b_max_mech = 2.5;   % decel max meccanica [m/s^2]


v_min_explore = 1.0;

% slip_warn = 0.15;
% slip_crit = 0.30;

a_long_reserve = 0.8;   % margine per longitudinal control [m/s^2]

%% Protezioni input
mu_next = max(mu_next, 0.05);
kappa_abs = max(abs(kappa_next), kappa_eps);

%% 1. Limite curva da friction circle
a_total_max = eta_mu * mu_next * g;
a_lat_allowed = sqrt(max(a_total_max^2 - a_long_reserve^2, 0));

v_curve_mu = sqrt(a_lat_allowed / kappa_abs);

%% 2. Limite anti-ribaltamento da geometria
a_y_roll_safe = eta_roll * g * T_track/(2*h_CG) - g*abs(sin(angle_lat));
a_y_roll_safe = max(a_y_roll_safe, 0.1);

v_rollover = sqrt(a_y_roll_safe / kappa_abs);

%% 3. Limite da spazio frenata
b_eff = eta_brake * mu_next * g * cos(angle_long) + g*sin(angle_long);
b_eff = min(b_eff, b_max_mech);
b_eff = max(b_eff, 0.2);

v_goal = sqrt(2*b_eff*max(d_goal - r_goal, 0));

%% 4. Limite da celle ignote
v_unknown = v_max_global * (1 - 0.6*unknown_ratio_ahead);
v_unknown = max(v_unknown, v_min_explore);

% %% 5. Limite da slip
% slip_max = max([abs(slip_FL), abs(slip_FR), abs(slip_RL), abs(slip_RR)]);
% 
% if slip_max > slip_crit
%     v_slip_safe = 0.5 * V;
% elseif slip_max > slip_warn
%     v_slip_safe = 0.8 * V;
% else
%     v_slip_safe = v_max_global;
% end

%% 6. Riduzione da LTR
Fz_left = Fz_FL + Fz_RL;
Fz_right = Fz_FR + Fz_RR;
LTR = abs(Fz_left - Fz_right) / max(Fz_left + Fz_right, 1e-6);

if LTR > 0.80
    v_ltr = 0.4 * V;
elseif LTR > 0.65
    v_ltr = 0.7 * V;
else
    v_ltr = v_max_global;
end

%% 7. Minimo finale
v_ref_raw = min([ ...
    v_max_global, ...
    v_rollover, ...
    v_goal, ...
    v_unknown, ...
    v_ltr]);

%% 8. Rate limiter solo in salita su v_ref
a_ref_up = 3.0;      % quanto rapidamente può salire v_ref [m/s^2]

% Primo step:
% v_ref_prev viene inizializzato a -1 nel blocco Unit Delay / Memory.
% Siccome v_ref non può mai essere negativo, -1 è un valore sentinella sicuro.
if v_ref_prev < 0
    v_ref = v_ref_raw;
else
    if v_ref_raw > v_ref_prev
        % La velocità di riferimento può salire gradualmente
        v_ref = min(v_ref_raw, v_ref_prev + a_ref_up*Ts);
    else
        % La velocità di riferimento può scendere immediatamente
        v_ref = v_ref_raw;
    end
end
%% 9. Saturazione finale
v_ref = min(max(v_ref, 0), v_max_global);
end

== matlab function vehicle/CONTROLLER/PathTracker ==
function [delta_cmd, kappa_next, dist_to_goal, goal_flag, e_cte, psi_e] = PathTracker( ...
    x, y, psi, vel, path_x, path_y, n_pts, K_y, K_psi, id, ranking)
%#codegen
%% Init output
delta_cmd    = 0.0;
kappa_next   = 0.0;
dist_to_goal = 999999; %perché se inizializzo piccolo è minore di r goal e potrebbero esserci problemi
goal_flag    = 0.0;
e_cte        = 0.0;
psi_e        = 0.0;
gx = 0.0;
gy = 0.0;
N = int32(n_pts);
if N < int32(3)
return;
end
%% Parametri veicolo
L_wb  = 1.5;
d_max = 0.56;
%% Parametri lookahead dinamico
Ld0    = 3.0;    % [m] lookahead minimo/base
kLd    = 0.5;    % [s] coefficiente velocità
Ld_min = 3.0;    % [m]
Ld_max = 12.0;   % [m]
Ld = Ld0 + kLd * abs(vel);
Ld = min(max(Ld, Ld_min), Ld_max);
%% Parametri deadband
e_dead     = 0.15;   % [m] errore laterale trascurabile
psi_dead   = 0.04;   % [rad] circa 2.3 gradi
kappa_dead = 0.01;   % [1/m] path quasi rettilineo
%% Trova il punto del path più vicino al veicolo
best_d2 = realmax;
best_i  = int32(2);
for i = int32(2):(N-int32(1))
    dx = path_x(i) - x;
    dy = path_y(i) - y;
    d2 = dx*dx + dy*dy;
if d2 < best_d2
        best_d2 = d2;
        best_i  = i;
end
end
%% Target point avanti lungo il path usando lookahead dinamico
target_i = best_i;
acc_dist = 0.0;
for i = best_i:(N-int32(1))
    dxp = path_x(i+1) - path_x(i);
    dyp = path_y(i+1) - path_y(i);
    ds  = sqrt(dxp*dxp + dyp*dyp);
    acc_dist = acc_dist + ds;
    target_i = i + int32(1);
if acc_dist >= Ld
break;
end
end
%% Protezione indici target
if target_i > N-int32(1)
    target_i = N-int32(1);
end
if target_i < int32(2)
    target_i = int32(2);
end
%% Heading del path usando il punto lookahead
dxh = path_x(target_i) - path_x(best_i);
dyh = path_y(target_i) - path_y(best_i);
if dxh*dxh + dyh*dyh > 1e-9
    path_heading = atan2(dyh, dxh);
else
    path_heading = atan2(path_y(best_i+1)-path_y(best_i-1), ...
                         path_x(best_i+1)-path_x(best_i-1));
end
%% Errore heading
psi_e = mod(path_heading - psi + pi, 2*pi) - pi;
%% Errore laterale
% Versore normale al path (comune ai due casi)
n_x = -sin(path_heading);
n_y =  cos(path_heading);

if id == ranking(1)
    % Veicolo LEADER (primo in classifica): l'e_cte viene proiettato sul
    % punto lookahead dinamico (target_i), cioè più avanti lungo il vettore
    % del path. Così il riferimento laterale non insegue i continui
    % replanning di A* e il controllo può convergere.
    xc = path_x(target_i);
    yc = path_y(target_i);
else
    % Tutti gli altri veicoli: e_cte sul closest point (comportamento attuale)
    xc = path_x(best_i);
    yc = path_y(best_i);
end

ex = x - xc;
ey = y - yc;
e_cte = ex*n_x + ey*n_y;
%% Curvatura media nei prossimi punti
lookahead_pts = int32(12);
last_i = min(N-int32(1), best_i + lookahead_pts);
kappa_sum     = 0.0;
kappa_count   = 0.0;
kappa_abs_max = 0.0;
for j = best_i:last_i
    xm = path_x(j-1); ym = path_y(j-1);
    xcj = path_x(j);  ycj = path_y(j);
    xp = path_x(j+1); yp = path_y(j+1);
    v1x = xcj - xm;
    v1y = ycj - ym;
    v2x = xp - xcj;
    v2y = yp - ycj;
    cross_z = v1x*v2y - v1y*v2x;
    a  = sqrt(v1x*v1x + v1y*v1y);
    b  = sqrt(v2x*v2x + v2y*v2y);
    cc = sqrt((xp-xm)^2 + (yp-ym)^2);
    denom = a*b*cc;
if denom > 1e-9
        kappa_j = (2.0 * abs(cross_z) / denom) * sign(cross_z);
else
        kappa_j = 0.0;
end
    kappa_sum = kappa_sum + kappa_j;
    kappa_count = kappa_count + 1.0;
if abs(kappa_j) > kappa_abs_max
        kappa_abs_max = abs(kappa_j);
end
end
if kappa_count > 0.0
    kappa_local = kappa_sum / kappa_count;
else
    kappa_local = 0.0;
end
% Per eventuale governor velocità: modulo massimo della curvatura futura
kappa_next = kappa_abs_max;
%% Feedforward di curvatura
if abs(kappa_local) < kappa_dead
    delta_ff = 0.0;
else
    delta_ff = atan(L_wb * kappa_local);
end
%% Feedback
delta_fb = -K_y * e_cte - K_psi * psi_e;
delta_cmd = delta_ff + delta_fb;
%% Deadband: se sei quasi dritto e vicino al path, sterzo zero
if abs(e_cte) < e_dead && abs(psi_e) < psi_dead && abs(kappa_local) < kappa_dead
    delta_cmd = 0.0;
end
%% Saturazione finale sterzo
delta_cmd = min(max(delta_cmd, -d_max), d_max);
%% Distanza dal goal
gx = path_x(N);
gy = path_y(N);
dist_to_goal = sqrt((gx - x)^2 + (gy - y)^2);
end

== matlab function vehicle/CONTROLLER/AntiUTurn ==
function [path_x_out, path_y_out, n_out, hold_flag, allow_uturn, long_rel, wait_s, mode] = ...
    PathRoleAntiUTurn(path_x_in, path_y_in, n_in, id, ranking, ValuesBus, Ts)
%PATHROLEANTIUTURN  (variante con un solo persistent struct)
% Stessa logica della versione precedente, ma tutto lo stato interno e'
% raccolto in un'unica struct persistente "st" -> piu' leggibile, stesso codegen.
%#codegen

%% ===================== PARAMETRI =======================================
MAX_PATH_LEN     = int32(1000);
BEHIND_MARGIN_M  = 1.0;
AHEAD_RELEASE_M  = 1.0;
GUARD_MAX_DIST_M = 8.0;
HOLD_AHEAD_M     = 6.0;
AWAY_TIME_S      = 2.0;
AHEAD_CONFIRM_S  = 0.3;
COOLDOWN_S       = 4.0;
DIST_INC_EPS     = 0.05;
V_LEADER_MIN     = 0.5;
T_WAIT_MAX_S     = 12.0;

if Ts <= 0
    Ts = 0.02;
end

AWAY_STEPS_REQ  = int32(ceil(AWAY_TIME_S    / Ts));
AHEAD_STEPS_REQ = int32(ceil(AHEAD_CONFIRM_S/ Ts));
COOLDOWN_STEPS  = int32(ceil(COOLDOWN_S     / Ts));

%% ===================== DEFAULT OUTPUT ==================================
path_x_out = path_x_in;
path_y_out = path_y_in;
n_out      = n_in;
hold_flag  = 0.0;
allow_uturn= 1.0;
long_rel   = 0.0;
wait_s     = 0.0;
mode       = 0.0;   % 0 pass-through, 1 hold, 2 released

%% ===================== ID / RANKING ====================================
my_id     = int32(id);
leader_id = int32(ranking(1));
is_leader = (my_id == leader_id);

%% ===================== STATO PERSISTENTE (unico) =======================
persistent st
if isempty(st)
    st = initState();
end

%% ===================== LEADER: PASS-THROUGH ============================
if is_leader
    st = resetGuard(st);          % azzera guard/contatori/cooldown
    st.prev_is_leader = true;
    st.prev_overshoot = false;
    st.initialized    = true;

    path_x_out = path_x_in;  path_y_out = path_y_in;  n_out = n_in;
    hold_flag  = 0.0;  allow_uturn = 1.0;  mode = 0.0;
    return;
end

%% ===================== STATO VEICOLO ===================================
[x, y, psi, ~] = readVehicleState(ValuesBus, my_id);
cpsi = cos(psi);
spsi = sin(psi);

%% ===================== GOAL ============================================
N = int32(round(n_in));
if N < int32(2);      N = int32(2);      end
if N > MAX_PATH_LEN;  N = MAX_PATH_LEN;  end

gx = path_x_in(N);  gy = path_y_in(N);
dx = gx - x;        dy = gy - y;
d_target = hypot(dx, dy);

long_rel = dx*cpsi + dy*spsi;   % solo output, non usato nelle decisioni

%% ===================== "DIETRO" RISPETTO AL PATH =======================
tnx = path_x_in(N) - path_x_in(N-1);
tny = path_y_in(N) - path_y_in(N-1);
tnorm = hypot(tnx, tny);
if tnorm < 1e-6
    tnx = cpsi;  tny = spsi;
else
    tnx = tnx / tnorm;  tny = tny / tnorm;
end

s_rel      = dx*tnx + dy*tny;
overshoot  = (s_rel < -BEHIND_MARGIN_M) && (d_target <= GUARD_MAX_DIST_M);
goal_ahead = (s_rel >  AHEAD_RELEASE_M);

%% ===================== ARMING ==========================================
just_demoted          = st.prev_is_leader && (~is_leader);
initial_follower_over = (~st.initialized) && overshoot;
overshoot_rising_edge = overshoot && (~st.prev_overshoot);

can_arm = (~st.guard_active) && (st.cooldown_count <= int32(0)) && overshoot;
should_start_guard = can_arm && ...
    (just_demoted || initial_follower_over || overshoot_rising_edge);

if should_start_guard
    st.guard_active = true;
    st.wait_count   = int32(0);
    st.away_count   = int32(0);
    st.ahead_count  = int32(0);
    st.last_dist    = d_target;

    [xL, yL, ~, vL] = readVehicleState(ValuesBus, leader_id);
    d_new_leader = hypot(xL - x, yL - y);
    t_min_wait = 2.0 * d_new_leader / max(abs(vL), V_LEADER_MIN);
    t_min_wait = min(t_min_wait, T_WAIT_MAX_S);
    st.min_wait_steps = int32(ceil(t_min_wait / Ts));
end

%% ===================== GUARD ATTIVO ====================================
if st.guard_active
    st.wait_count = st.wait_count + int32(1);

    if d_target > st.last_dist + DIST_INC_EPS
        st.away_count = st.away_count + int32(1);
    else
        st.away_count = int32(0);
    end

    if goal_ahead
        st.ahead_count = st.ahead_count + int32(1);
    else
        st.ahead_count = int32(0);
    end

    waited_enough   = st.wait_count  >= st.min_wait_steps;
    away_for_2s     = st.away_count  >= AWAY_STEPS_REQ;
    ahead_confirmed = st.ahead_count >= AHEAD_STEPS_REQ;

    release_guard = ahead_confirmed || waited_enough || away_for_2s;

    if release_guard
        st.guard_active   = false;
        st.cooldown_count = COOLDOWN_STEPS;

        path_x_out = path_x_in;  path_y_out = path_y_in;  n_out = n_in;
        hold_flag  = 0.0;  allow_uturn = 1.0;  mode = 2.0;
    else
        path_x_out = zeros(size(path_x_in));
        path_y_out = zeros(size(path_y_in));
        path_x_out(1) = x;                       path_y_out(1) = y;
        path_x_out(2) = x + HOLD_AHEAD_M * cpsi;  path_y_out(2) = y + HOLD_AHEAD_M * spsi;
        n_out = 2.0;

        hold_flag  = 1.0;  allow_uturn = 0.0;  mode = 1.0;
    end

    st.last_dist = d_target;

else
    if st.cooldown_count > int32(0)
        st.cooldown_count = st.cooldown_count - int32(1);
    end
end

%% ===================== UPDATE MEMORIA ==================================
wait_s = double(st.wait_count) * Ts;
st.prev_is_leader = is_leader;
st.prev_overshoot = overshoot;
st.initialized    = true;

end

%% ========================================================================
function st = initState()
%#codegen
st.initialized    = false;
st.prev_is_leader = false;
st.prev_overshoot = false;
st.guard_active   = false;
st.wait_count     = int32(0);
st.away_count     = int32(0);
st.ahead_count    = int32(0);
st.cooldown_count = int32(0);
st.last_dist      = 0.0;
st.min_wait_steps = int32(0);
end

%% ========================================================================
function st = resetGuard(st)
%#codegen
st.guard_active   = false;
st.wait_count     = int32(0);
st.away_count     = int32(0);
st.ahead_count    = int32(0);
st.cooldown_count = int32(0);
end

%% ========================================================================
function [x, y, psi, v] = readVehicleState(ValuesBus, id)
%#codegen
if int32(id) == int32(1)
    x = ValuesBus.id1.x;  y = ValuesBus.id1.y;
    psi = ValuesBus.id1.psi; v = ValuesBus.id1.vel_totale;
elseif int32(id) == int32(2)
    x = ValuesBus.id2.x;  y = ValuesBus.id2.y;
    psi = ValuesBus.id2.psi; v = ValuesBus.id2.vel_totale;
else
    x = ValuesBus.id3.x;  y = ValuesBus.id3.y;
    psi = ValuesBus.id3.psi; v = ValuesBus.id3.vel_totale;
end
end





% function [path_x_out, path_y_out, n_out, hold_flag, allow_uturn, long_rel, wait_s, mode] = ...
%     PathRoleAntiUTurn(path_x_in, path_y_in, n_in, id, ranking, ValuesBus, Ts)
% %PATHROLEANTIUTURN
% % Filtro path prima del PathTracker.
% %
% % Obiettivo:
% % - se il veicolo e' leader: lascia passare il path originale;
% % - se e' follower e il target e' dietro: evita inversione a U immediata;
% % - aspetta che il target passi davanti oppure che sia chiaro che si sta
% %   allontanando.
% %
% %#codegen
% 
% %% ===================== PARAMETRI =======================================
% 
% MAX_PATH_LEN = int32(1000);
% 
% % Target considerato "dietro" solo se sta almeno 2 m dietro al veicolo
% BEHIND_MARGIN_M = 2.0;
% 
% % Rilascio normale quando il target passa almeno 2 m davanti
% AHEAD_RELEASE_M = 2.0;
% 
% % Path fittizio davanti al veicolo mentre si aspetta.
% % Deve essere > r_goal se vuoi evitare che il PathTracker lo consideri
% % subito raggiunto. Nel tuo scenario r_goal e' circa 5 m.
% HOLD_AHEAD_M = 6.0;
% 
% % Tempo minimo per dire: "il target si sta allontanando"
% AWAY_TIME_S = 2.0;
% 
% % Incremento minimo distanza target per contare come allontanamento
% DIST_INC_EPS = 0.05;
% 
% % Velocita' minima leader per evitare divisioni per zero
% V_LEADER_MIN = 0.5;
% 
% % Safety cap: evita attese infinite se il leader e' molto lento.
% % Se vuoi rispettare rigidamente la tua formula, alza molto questo valore.
% T_WAIT_MAX_S = 12.0;
% 
% % Safety sample time
% if Ts <= 0
%     Ts = 0.02;
% end
% 
% AWAY_STEPS_REQ = int32(ceil(AWAY_TIME_S / Ts));
% 
% %% ===================== DEFAULT OUTPUT ==================================
% 
% path_x_out = path_x_in;
% path_y_out = path_y_in;
% n_out      = n_in;
% 
% hold_flag   = 0.0;
% allow_uturn = 1.0;
% long_rel    = 0.0;
% wait_s      = 0.0;
% mode        = 0.0;   % 0 pass-through, 1 hold, 2 released
% 
% %% ===================== LETTURA ID/RANKING ===============================
% 
% my_id     = int32(id);
% leader_id = int32(ranking(1));
% 
% is_leader = (my_id == leader_id);
% 
% %% ===================== PERSISTENT ======================================
% 
% persistent initialized
% persistent prev_is_leader
% persistent prev_target_behind
% persistent guard_active
% persistent wait_count
% persistent away_count
% persistent last_dist
% persistent min_wait_steps
% 
% if isempty(initialized)
%     initialized        = false;
%     prev_is_leader     = false;
%     prev_target_behind = false;
%     guard_active       = false;
%     wait_count         = int32(0);
%     away_count         = int32(0);
%     last_dist          = 0.0;
%     min_wait_steps     = int32(0);
% end
% 
% %% ===================== SE SONO LEADER: PASSO TUTTO ======================
% 
% if is_leader
%     guard_active       = false;
%     wait_count         = int32(0);
%     away_count         = int32(0);
%     prev_is_leader     = true;
%     prev_target_behind = false;
%     initialized        = true;
% 
%     path_x_out = path_x_in;
%     path_y_out = path_y_in;
%     n_out      = n_in;
% 
%     hold_flag   = 0.0;
%     allow_uturn = 1.0;
%     wait_s      = 0.0;
%     mode        = 0.0;
%     return;
% end
% 
% %% ===================== LETTURA STATO VEICOLO ============================
% 
% [x, y, psi, ~] = readVehicleState(ValuesBus, my_id);
% 
% %% ===================== TARGET = ULTIMO PUNTO DEL PATH ===================
% 
% N = int32(round(n_in));
% 
% if N < int32(2)
%     N = int32(2);
% end
% 
% if N > MAX_PATH_LEN
%     N = MAX_PATH_LEN;
% end
% 
% tx = path_x_in(N);
% ty = path_y_in(N);
% 
% dx = tx - x;
% dy = ty - y;
% 
% cpsi = cos(psi);
% spsi = sin(psi);
% 
% % Proiezione longitudinale del target nel frame veicolo
% long_rel = dx*cpsi + dy*spsi;
% 
% target_behind = long_rel < -BEHIND_MARGIN_M;
% target_ahead  = long_rel >  AHEAD_RELEASE_M;
% 
% d_target = hypot(dx, dy);
% 
% %% ===================== EVENTI DI ATTIVAZIONE GUARD ======================
% 
% just_demoted = prev_is_leader && ~is_leader;
% 
% % Serve soprattutto per le condizioni iniziali random:
% % se il blocco parte gia' da follower con target dietro, attivo il guard.
% initial_follower_behind = (~initialized) && (~is_leader) && target_behind;
% 
% % Serve se un follower normale supera il proprio target e questo gli finisce dietro.
% target_just_went_behind = target_behind && (~prev_target_behind);
% 
% should_start_guard = ...
%     (~guard_active) && ...
%     target_behind && ...
%     (just_demoted || initial_follower_behind || target_just_went_behind);
% 
% if should_start_guard
% 
%     guard_active = true;
%     wait_count   = int32(0);
%     away_count   = int32(0);
%     last_dist    = d_target;
% 
%     % Lettura nuovo leader
%     [xL, yL, ~, vL] = readVehicleState(ValuesBus, leader_id);
% 
%     d_new_leader = hypot(xL - x, yL - y);
% 
%     % Tua logica:
%     % tempo attesa = 2 * distanza nuovo leader / velocita nuovo leader
%     t_min_wait = 2.0 * d_new_leader / max(abs(vL), V_LEADER_MIN);
% 
%     % Safety: evita blocco infinito con leader fermo/lento
%     t_min_wait = min(t_min_wait, T_WAIT_MAX_S);
% 
%     min_wait_steps = int32(ceil(t_min_wait / Ts));
% end
% 
% %% ===================== MODALITA' GUARD ACTIVE ===========================
% 
% if guard_active
% 
%     wait_count = wait_count + int32(1);
% 
%     % Ricontrollo distanza corrente dal target
%     d_target_now = d_target;
% 
%     % Conta solo aumenti consecutivi della distanza
%     if d_target_now > last_dist + DIST_INC_EPS
%         away_count = away_count + int32(1);
%     else
%         away_count = int32(0);
%     end
% 
%     waited_enough      = wait_count >= min_wait_steps;
%     target_away_for_2s = away_count >= AWAY_STEPS_REQ;
% 
%     % Condizioni di rilascio:
%     % 1) il target e' passato davanti;
%     % 2) ho aspettato il tempo stimato;
%     % 3) il target si sta allontanando da almeno 2 secondi.
%     release_guard = target_ahead || waited_enough || target_away_for_2s;
% 
%     if release_guard
% 
%         guard_active = false;
% 
%         path_x_out = path_x_in;
%         path_y_out = path_y_in;
%         n_out      = n_in;
% 
%         hold_flag   = 0.0;
%         allow_uturn = 1.0;
%         mode        = 2.0;
% 
%     else
% 
%         % HOLD:
%         % Non mando al tracker il target dietro.
%         % Gli mando un micro-path davanti al veicolo, così non comanda U-turn.
%         path_x_out = zeros(size(path_x_in));
%         path_y_out = zeros(size(path_y_in));
% 
%         path_x_out(1) = x;
%         path_y_out(1) = y;
% 
%         path_x_out(2) = x + HOLD_AHEAD_M * cpsi;
%         path_y_out(2) = y + HOLD_AHEAD_M * spsi;
% 
%         n_out = 2.0;
% 
%         hold_flag   = 1.0;
%         allow_uturn = 0.0;
%         mode        = 1.0;
%     end
% 
%     last_dist = d_target_now;
% end
% 
% %% ===================== UPDATE MEMORIA ==================================
% 
% wait_s = double(wait_count) * Ts;
% 
% prev_is_leader     = is_leader;
% prev_target_behind = target_behind;
% initialized        = true;
% 
% end
% 
% %% ========================================================================
% function [x, y, psi, v] = readVehicleState(ValuesBus, id)
% % Lettura statica codegen-friendly dal bus.
% 
% if int32(id) == int32(1)
% 
%     x   = ValuesBus.id1.x;
%     y   = ValuesBus.id1.y;
%     psi = ValuesBus.id1.psi;
%     v   = ValuesBus.id1.vel_totale;
% 
% elseif int32(id) == int32(2)
% 
%     x   = ValuesBus.id2.x;
%     y   = ValuesBus.id2.y;
%     psi = ValuesBus.id2.psi;
%     v   = ValuesBus.id2.vel_totale;
% 
% else
% 
%     x   = ValuesBus.id3.x;
%     y   = ValuesBus.id3.y;
%     psi = ValuesBus.id3.psi;
%     v   = ValuesBus.id3.vel_totale;
% 
% end
% 
% end

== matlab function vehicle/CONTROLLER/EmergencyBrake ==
function obs_flag = ObstacleBrakeFlag(x, y, psi, vel)
%OBSTACLEBRAKEFLAG Wrapper Simulink per emergency brake, con HOLD di rilascio.
% Anche quando il pericolo finisce, mantiene il flag a 1 per HOLD_STEPS passi
% (il blocco gira a dtastar = 0.1 s, quindi 5 passi = 0.5 s) per togliere
% lo sfarfallio del flag al bordo del pericolo.
%#codegen

coder.extrinsic('obstacle_brake_from_base');

HOLD_STEPS = int32(5);   % passi di mantenimento dopo fine pericolo (0.1 s per passo)

persistent hold_cnt
if isempty(hold_cnt)
    hold_cnt = int32(0);
end

tmp = 0.0;
tmp = obstacle_brake_from_base(x, y, psi, vel);
raw = double(tmp);

if raw >= 0.5
    hold_cnt = HOLD_STEPS;            % pericolo presente: arma il mantenimento
    obs_flag = 1.0;
elseif hold_cnt > int32(0)
    hold_cnt = hold_cnt - int32(1);   % pericolo finito: continua a frenare nel hold
    obs_flag = 1.0;
else
    obs_flag = 0.0;
end

end

== matlab function vehicle/PLANT/VEHICLE 8DOF/Dinamica Rotazionale 
Ruote (EBD & ABS)/ABS/ABS_Logic ==
function [target, flag] = ABS_logic(brakes_in, slip, last_brake)
% ABS fittizio - logica vettoriale (una riga per ruota).
%
%   Ingressi: vettori Nx1  (tipicamente N=4)
%     brakes_in  : richiesta freno [%] non corretta
%     slip       : slip ruota [-]  (< 0 = bloccaggio)
%     last_brake : uscita ciclo precedente (feedback via Memory)
%
%   Uscite: vettori Nx1
%     target : richiesta corretta [%]
%     flag   : 0=OFF, 1=HOLD, 2=RELEASE  (uint8)

slip_release = -0.20;
slip_hold    = -0.12;

n      = numel(slip);
target = zeros(n, 1);
flag   = zeros(n, 1, 'uint8');

for i = 1:n
    if slip(i) <= slip_release
        target(i) = 0;
        flag(i)   = uint8(2);
    elseif slip(i) <= slip_hold
        target(i) = last_brake(i);
        flag(i)   = uint8(1);
    else
        target(i) = brakes_in(i);
        flag(i)   = uint8(0);
    end
end
